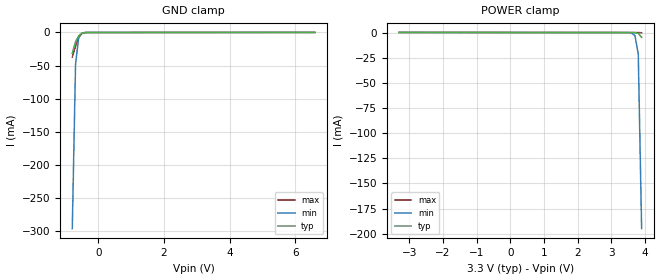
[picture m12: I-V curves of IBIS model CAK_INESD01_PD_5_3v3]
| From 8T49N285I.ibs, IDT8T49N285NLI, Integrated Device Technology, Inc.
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[Model] CAK_INESD01_PD_5_3v3
Model_type   Input
Polarity   Non-Inverting
Vinl = 0.8V
Vinh = 2.0V
|   typ   min   max
C_comp   2pF   1.5pF   2.5pF
|   typ   min   max
[Voltage range]   3.3V   3.135V   3.465V
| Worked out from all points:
|   GND clamp passes 1 mA (typ) near -0.51 V on its own axis
[GND_clamp]
|Voltage   I (typ)   I (min)   I (max)
|Note, modeling breaks down at 250mA and above.  This is well beyond the functional   |
|operating range of the device.  Should this scenario occur, catastrophic failure and   |
|possible damage to the device and/or board is of higher concern than the I-V curve   |
|behavior.  The IBIS checker will flag currents in excess of 10A with warnings.  Lines   |
|with currents in excess of 0.35 A have been commented out.  The points still remain|
|available to the user if the user desires to use them.   |
|-3.30000e+00   -9.36883e+00   -7.41795e+00   -1.15553e+01
|-3.20000e+00   -8.98673e+00   -7.13120e+00   -1.10681e+01
|-3.10000e+00   -8.60465e+00   -6.84454e+00   -1.05809e+01
|-3.00000e+00   -8.22259e+00   -6.55796e+00   -1.00937e+01
|-2.90000e+00   -7.84055e+00   -6.27147e+00   -9.60644e+00
|-2.80000e+00   -7.45854e+00   -5.98508e+00   -9.11917e+00
|-2.70000e+00   -7.07656e+00   -5.69880e+00   -8.63189e+00
|-2.60000e+00   -6.69464e+00   -5.41263e+00   -8.14461e+00
|-2.50000e+00   -6.31277e+00   -5.12658e+00   -7.65734e+00
|-2.40000e+00   -5.93098e+00   -4.84067e+00   -7.17007e+00
|-2.30000e+00   -5.54926e+00   -4.55490e+00   -6.68283e+00
|-2.20000e+00   -5.16764e+00   -4.26929e+00   -6.19563e+00
|-2.10000e+00   -4.78614e+00   -3.98385e+00   -5.70849e+00
|-2.00000e+00   -4.40478e+00   -3.69859e+00   -5.22142e+00
|-1.90000e+00   -4.02357e+00   -3.41352e+00   -4.73446e+00
|-1.80000e+00   -3.64255e+00   -3.12867e+00   -4.24763e+00
|-1.70000e+00   -3.26174e+00   -2.84405e+00   -3.76095e+00
|-1.60000e+00   -2.88119e+00   -2.55967e+00   -3.27445e+00
|-1.50000e+00   -2.50093e+00   -2.27556e+00   -2.78816e+00
|-1.40000e+00   -2.12099e+00   -1.99172e+00   -2.30213e+00
|-1.30000e+00   -1.74144e+00   -1.70816e+00   -1.81643e+00
|-1.20000e+00   -1.36232e+00   -1.42492e+00   -1.33112e+00
|-1.10000e+00   -9.83665e-01   -1.14201e+00   -8.46289e-01
|-1.00000e+00   -6.05544e-01   -8.59493e-01   -3.62030e-01
|-9.00000e-01   -2.28020e-01   -5.77510e-01   -5.71068e-02
-800mV    -31.51mA   -296.3mA   -37.05mA
-700mV    -13.96mA   -47.9mA    -20.78mA
-600mV    -4.826mA   -5.935mA   -7.491mA
-500mV    -779.4uA   -884.9uA   -1.121mA
-300mV    -7.644uA   -12.06uA   -7.746uA
6.6V      131.5uA    115.2uA    151.9uA
[Power_clamp]
|Voltage   I (typ)   I (min)   I (max)
|Note, modeling breaks down at 250mA and above.  This is well beyond the functional   |
|operating range of the device.  Should this scenario occur, catastrophic failure and   |
|possible damage to the device and/or board is of higher concern than the I-V curve   |
|behavior.  The IBIS checker will flag currents in excess of 10A with warnings.  Lines   |
|with currents in excess of 0.35 A have been commented out.  The points still remain|
|available to the user if the user desires to use them.   |
-3.3V     131.5uA    112.4uA    155.7uA
3.5V      -4.021uA   -43.46uA   -805.9nA
3.6V      -7.644uA   -413.5uA   -3.108uA
3.7V      -58.35uA   -3.051mA   -5.447uA
3.8V      -779.4uA   -21.2mA    -11.73uA
3.9V      -4.826mA   -194.9mA   -182.9uA
